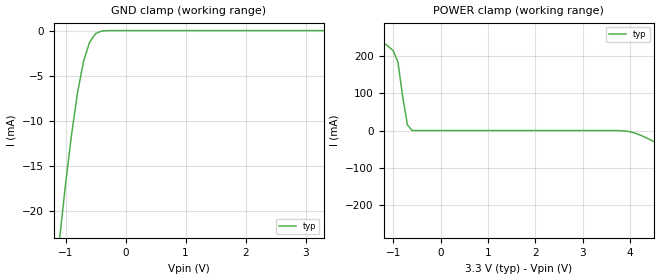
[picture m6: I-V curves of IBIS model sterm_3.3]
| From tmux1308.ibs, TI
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| sterm_3.3
[Model]   sterm_3.3
Model_type   Terminator
|   typ   min   max
C_comp   1.008417e-12   NA   NA
[Voltage Range]   3.3   NA   NA
[Temperature Range]   27   NA   NA
[Power Clamp Reference]   3.3   NA   NA
[GND Clamp Reference]   0   NA   NA
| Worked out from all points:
|   GND clamp passes 1 mA (typ) near -0.57 V on its own axis
|   POWER clamp passes 1 mA (typ) near -0.61 V on its own axis
[GND Clamp]
|   Voltage   I(typ)   I(min)   I(max)
-6.6V     -37.87kA   NA         NA
-1.1V     -23.15mA   NA         NA
-1V       -17.04mA   NA         NA
-900mV    -11.54mA   NA         NA
-800mV    -6.888mA   NA         NA
-700mV    -3.398mA   NA         NA
-600mV    -1.315mA   NA         NA
-500mV    -338.5uA   NA         NA
-400mV    -44.29uA   NA         NA
-300mV    -3.116uA   NA         NA
3.3V      1.528nA    NA         NA
[POWER Clamp]
|   Voltage   I(typ)   I(min)   I(max)
-3.3V     428.2mA    NA         NA
-1.7V     280.6mA    NA         NA
-1.1V     226.6mA    NA         NA
-900mV    184.4mA    NA         NA
-700mV    15.37mA    NA         NA
-600mV    61.75uA    NA         NA
3.8V      -338.5uA   NA         NA
4.3V      -17.04mA   NA         NA
6.2V      -170.7mA   NA         NA
6.3V      -249.2mA   NA         NA
6.4V      -3.114A    NA         NA
6.6V      -1.138kA   NA         NA
